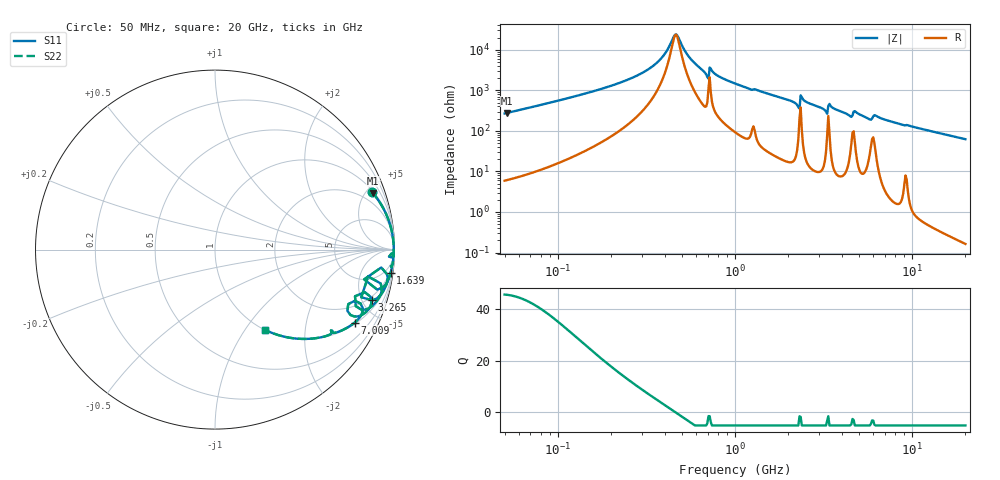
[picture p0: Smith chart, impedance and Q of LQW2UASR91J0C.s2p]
!Murata Part Number: LQW2UASR91J0C
!These Parameters are Measured in Series Mode Connection
!  o--[Z]--o
!Port1  Port2
!  o-------o
!Freq. Start=50[MHz] Stop=20[GHz], 401[Steps]
# Hz S RI R 50
!Freq.(Hz) S11(Real) S11(Imag) S21(Real) S21(Imag) S12(Real) S12(Imag) S22(Real) S22(Imag)
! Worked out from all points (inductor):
!   401 points, 50 MHz to 20 GHz, reference 50 ohm
!   read as one part in series: L = 844 nH near 51.52 MHz
!   highest Q = 45.4 at 51.52 MHz (marker M1), where L = 856 nH
!   self-resonance near 458.9 MHz
!   S11 on the Smith chart (normalised r, x): 50 MHz: 1.12, +5.37; 1.639 GHz: 2, -15; 3.265 GHz: 1.60, -5.93; 7.009 GHz: 1.07, -3.80; 20 GHz: 1.00, -1.25
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5e7  0.873 0.3222  0.127 -0.3222  0.127 -0.3222  0.873 0.3222
5.152053e7  0.8794 0.3149  0.1206 -0.3149  0.1206 -0.3149  0.8794 0.3149
1.364002e8  0.9799 0.1232  0.0201 -0.1232  0.0201 -0.1232  0.9799 0.1232
2.597386e8  0.9933 0.0494  0.00668 -0.0494  0.00668 -0.0494  0.9933 0.0494
3.721004e8  0.9955 0.018  0.00448 -0.018  0.00448 -0.018  0.9955 0.018
4.658406e8  0.9959 -0.000403  0.00414 0.000403  0.00414 0.000403  0.9959 -0.000403
5.492803e8  0.9956 -0.0141  0.00436 0.0141  0.00436 0.0141  0.9956 -0.0141
6.87656e8  0.9919 -0.0394  0.00811 0.0394  0.00811 0.0394  0.9919 -0.0394
7.411344e8  0.9933 -0.032  0.00668 0.032  0.00668 0.032  0.9933 -0.032
1e9  0.9913 -0.0667  0.00872 0.0667  0.00872 0.0667  0.9913 -0.0667
1.639343e9  0.9788 -0.1283  0.0212 0.1283  0.0212 0.1283  0.9788 -0.1283
2.245319e9  0.9347 -0.2108  0.0653 0.2108  0.0653 0.2108  0.9347 -0.2108
2.419936e9  0.9617 -0.1569  0.0383 0.1569  0.0383 0.1569  0.9617 -0.1569
2.728004e9  0.9481 -0.2098  0.0519 0.2098  0.0519 0.2098  0.9481 -0.2098
3.265178e9  0.876 -0.2828  0.124 0.2828  0.124 0.2828  0.876 -0.2828
3.466789e9  0.9295 -0.2195  0.0705 0.2195  0.0705 0.2195  0.9295 -0.2195
4.405649e9  0.8371 -0.3341  0.1629 0.3341  0.1629 0.3341  0.8371 -0.3341
4.81993e9  0.8722 -0.2875  0.1278 0.2875  0.1278 0.2875  0.8722 -0.2875
5.598765e9  0.7926 -0.3724  0.2074 0.3724  0.2074 0.3724  0.7926 -0.3724
7.009217e9  0.7787 -0.4062  0.2213 0.4062  0.2213 0.4062  0.7787 -0.4062
7.442007e9  0.7517 -0.4257  0.2483 0.4257  0.2483 0.4257  0.7517 -0.4257
2e10  0.2811 -0.4482  0.7189 0.4482  0.7189 0.4482  0.2811 -0.4482
